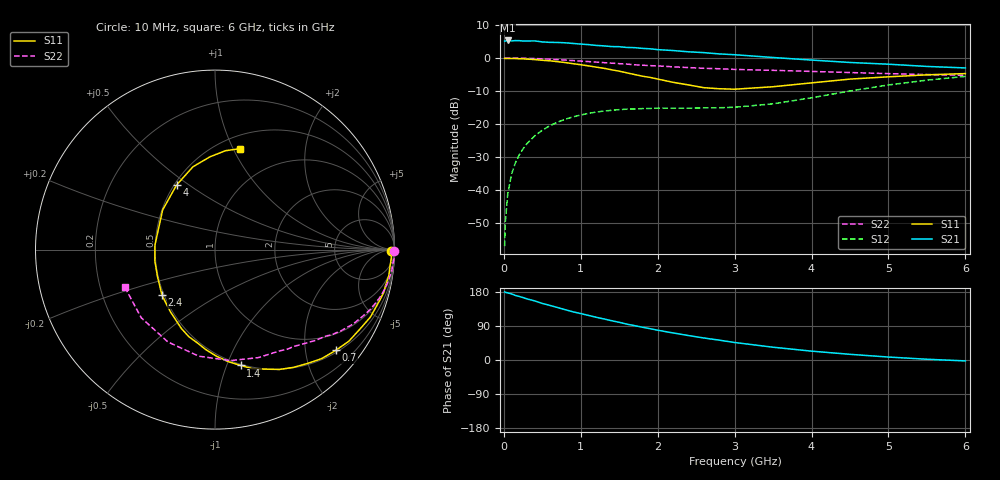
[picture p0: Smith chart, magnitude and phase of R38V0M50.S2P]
! SIEMENS Small Signal Semiconductors
! BFR181
! Si NPN RF Bipolar Junction Transistor in SOT23
! VCE = 8 V  IC = 0.5 mA
! Common Emitter S-Parameters:  May  1996
# GHz  S  MA  R  50
!  f  S11  S21  S12  S22
! GHz  MAG  ANG  MAG  ANG  MAG  ANG  MAG  ANG
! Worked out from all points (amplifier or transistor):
!   36 points, 10 MHz to 6 GHz, reference 50 ohm
!   highest |S21| = 5.3 dB at 50 MHz (marker M1)
!   |S21| within 3 dB of that: start of sweep to 2.158 GHz
!   unconditionally stable (mu >= 1): 2.4 GHz to 3.971 GHz
!   at 250 MHz: K = 0.12, MSG = 16.3 dB, |S12| = -27.6 dB
!   at 1.4 GHz: K = 0.60, MSG = 9.7 dB, |S12| = -15.9 dB
!   at 6 GHz: K = 0.92, MSG = 1.3 dB, |S12| = -5.6 dB
!   S11 on the Smith chart (normalised r, x): 10 MHz: open; 700 MHz: 0.55, -2.67; 1.4 GHz: 0.49, -1.12; 2.4 GHz: 0.49, -0.29; 4 GHz: 0.51, +0.45; 6 GHz: 0.63, +1.06
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0.01  0.9829 -0.5  1.8 179.7  0.0014 98.5  0.9996 -0.3
0.02  0.9828 -1.2  1.807 178.6  0.0033 91.3  0.9955 -0.6
0.05  0.9837 -2.7  1.84 177.2  0.0085 86.2  0.999 -1.4
0.1  0.9794 -5.5  1.809 174.4  0.0172 85.4  0.9996 -2.8
0.15  0.9794 -8.6  1.831 170.4  0.0257 84.0  0.9949 -4.2
0.25  0.9699 -14.4  1.801 164.7  0.0418 79.2  0.9916 -7.0
0.4  0.9441 -23.4  1.812 156.0  0.0657 74.0  0.9787 -11.1
0.5  0.9215 -28.6  1.749 149.3  0.08 69.9  0.968 -13.7
0.7  0.877 -39.7  1.716 138.3  0.1064 62.8  0.9418 -18.6
0.9  0.8173 -50.9  1.658 127.1  0.1278 56.0  0.9112 -23.2
1.1  0.7577 -61.8  1.592 117.7  0.1443 50.4  0.8801 -27.4
1.4  0.6612 -77.5  1.486 103.7  0.1605 43.2  0.834 -33.0
1.7  0.5598 -95.2  1.432 90.7  0.1682 38.6  0.7869 -37.6
2.2  0.4267 -125.6  1.294 71.4  0.1725 34.8  0.7328 -44.9
2.4  0.3899 -139.2  1.238 64.5  0.1726 35.1  0.714 -47.8
3  0.3355 175.7  1.118 46.2  0.1787 40.5  0.6696 -57.4
3.5  0.3658 142.9  1.015 33.7  0.2014 46.9  0.6484 -68.2
4  0.4185 120.8  0.928 23.4  0.2486 51.4  0.6243 -82.1
4.5  0.4776 104.9  0.853 15.0  0.3152 50.4  0.6007 -98.6
5  0.5173 93.2  0.803 7.8  0.3893 45.6  0.5777 -117.0
5.5  0.5539 84.0  0.743 2.0  0.4604 38.4  0.5596 -137.2
6  0.5791 76.1  0.705 -2.4  0.524 29.7  0.5443 -157.2
